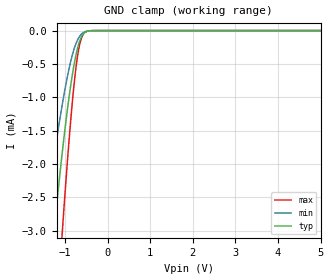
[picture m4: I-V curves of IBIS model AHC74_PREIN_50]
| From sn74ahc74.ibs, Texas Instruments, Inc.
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[Model]   AHC74_PREIN_50
Model_type  Input
Vinl= 1.65
Vinh= 3.85
| variable   typ   min   max
C_comp   0.69pF   0.59pF   0.79pF
[Temperature Range]   40   100   -40
| Ambient temperature   25   85   -40
[Voltage range]   5   4.5   5.5
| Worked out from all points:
|   GND clamp passes 1 mA (typ) near -0.91 V on its own axis
[GND Clamp]
| AHC74_PREIN_50
|   Voltage   I(typ)   I(min)   I(max)
-5V       -39.11mA   -25.77mA   -50.08mA
-1.5V     -4.697mA   -2.999mA   -7.43mA
-1.27V    -3.086mA   -1.94mA    -5.015mA
-1.245V   -2.922mA   -1.832mA   -4.762mA
-1.07V    -1.853mA   -1.126mA   -3.066mA
-1.05V    -1.74mA    -1.052mA   -2.883mA
-875mV    -857.1uA   -483.9uA   -1.406mA
-765mV    -433uA     -232.5uA   -670.7uA
-665mV    -173.1uA   -93.8uA    -234.3uA
-615mV    -93.6uA    -53.56uA   -114.5uA
-545mV    -32.78uA   -20.83uA   -33.46uA
5V        15.07nA    1.006nA    138.2nA
